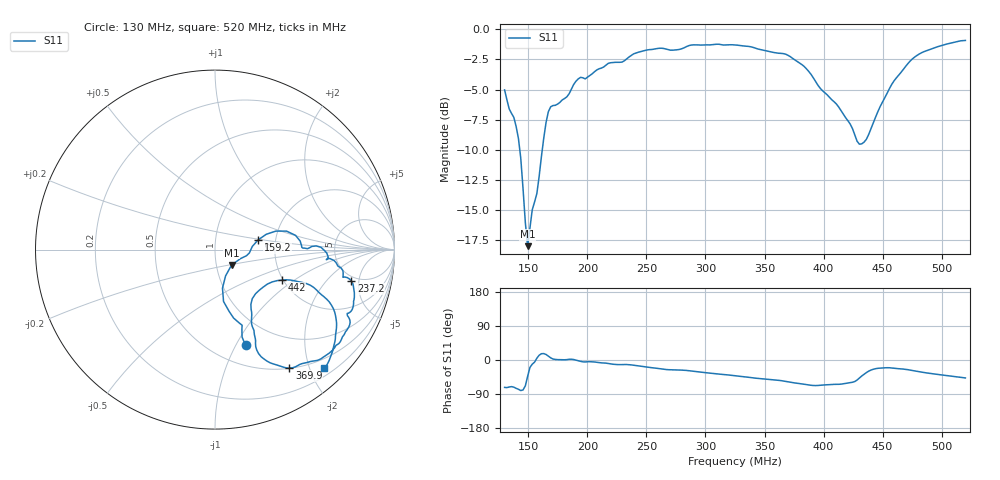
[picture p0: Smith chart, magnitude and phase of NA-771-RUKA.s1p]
!Agilent N9912A: A.05.34
!Date: Friday, 14 June 2013 16:45:03
!Model: N9912A
!Serial: MY50492702
!CABLE_LOSS: 0.000
!CABLE_NAME:
!VELOCITY_FACTOR: 1.000000000
!GPS Latitude:
!GPS Longitude:
!GPS TimeStamp: 0001-01-01 00:00:00Z
!GPS Seconds Since Last Read: 0
!CHECKSUM:1611618412
!Correction: S11(ON*)
!S1P File: Measurement: S11:
# Hz S DB R 50
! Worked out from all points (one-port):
!   201 points, 130 MHz to 520 MHz, reference 50 ohm
!   lowest |S11| = -18.0 dB at 149.5 MHz (marker M1), VSWR 1.29, Z = 59.2 - j10.4 ohm
!   |S11| at or under -10 dB: 142.8 MHz to 161.9 MHz (19.03 MHz wide, 12.5 % of centre)
!   S11 on the Smith chart (normalised r, x): 130 MHz: 0.70, -1.10; 159.2 MHz: 1.62, +0.19; 237.2 MHz: 4.45, -3.94; 369.9 MHz: 0.50, -1.70; 442 MHz: 1.97, -0.80; 520 MHz: 0.33, -2.24
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1.3e8  -5.03 -72.3
1.417e8  -9.06 -77.1
1.456e8  -13.21 -79.0
1.495e8  -17.98 -43.1
1.534e8  -14.96 -11.0
1.5925e8  -12.18 12.7
1.6315e8  -9.01 16.9
1.6705e8  -6.83 10.0
1.7095e8  -6.33 2.6
1.7875e8  -5.86 0.7
1.8655e8  -4.97 2.1
1.924e8  -4.11 -1.8
2.275e8  -2.74 -12.2
2.3725e8  -2.17 -12.9
2.6455e8  -1.60 -24.4
2.7625e8  -1.70 -26.3
2.8795e8  -1.32 -29.2
3.25e8  -1.31 -41.6
3.6985e8  -2.16 -57.9
3.7375e8  -2.42 -59.9
3.9325e8  -4.35 -67.4
4.225e8  -7.86 -59.7
4.303e8  -9.53 -47.4
4.42e8  -7.76 -24.5
4.5565e8  -4.93 -20.5
4.7125e8  -2.86 -25.5
4.927e8  -1.58 -36.4
5.2e8  -0.93 -47.3
